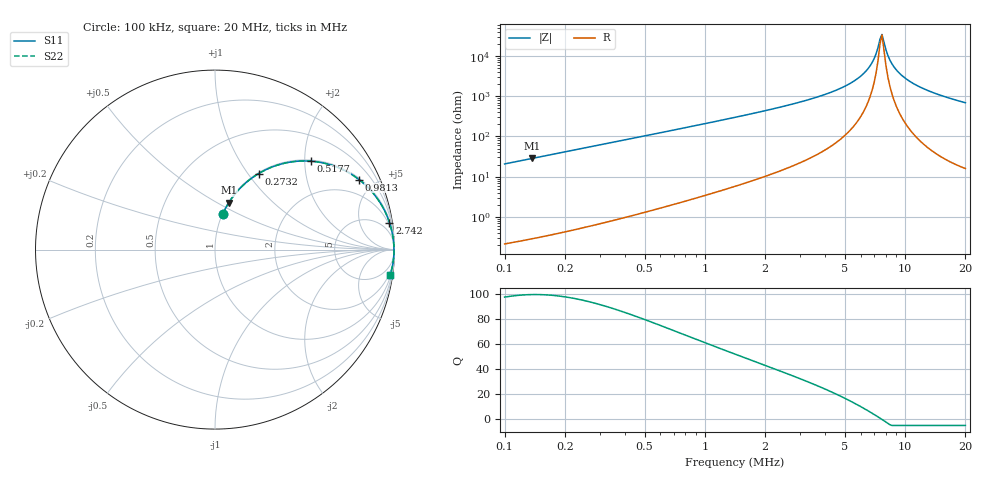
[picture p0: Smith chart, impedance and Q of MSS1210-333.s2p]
# MHz S MA R 50
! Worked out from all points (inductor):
!   233 points, 100 kHz to 20 MHz, reference 50 ohm
!   read as one part in series: L = 33 uH near 102.3 kHz
!   highest Q = 99.7 at 137.7 kHz (marker M1), where L = 32.9 uH
!   self-resonance near 7.491 MHz
!   S11 on the Smith chart (normalised r, x): 100 kHz: 1.00, +0.41; 273.2 kHz: 1.01, +1.13; 517.7 kHz: 1.03, +2.14; 981.3 kHz: 1.07, +4.08; 2.742 MHz: 1, +13; 20 MHz: 1, -14
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0.1  0.2027 77.7  0.9772 -11.7  0.9772 -11.7  0.2027 77.7
0.1376751  0.2734 73.6  0.9592 -15.9  0.9592 -15.9  0.2734 73.6
0.2436751  0.4476 62.8  0.8895 -26.6  0.8895 -26.6  0.4476 62.8
0.2731507  0.4889 60.1  0.8671 -29.3  0.8671 -29.3  0.4889 60.1
0.5177412  0.7255 42.8  0.6791 -46.5  0.6791 -46.5  0.7255 42.8
0.5937753  0.7699 38.9  0.628 -50.3  0.628 -50.3  0.7699 38.9
0.9813485  0.8924 25.9  0.437 -63.2  0.437 -63.2  0.8924 25.9
1.446882  0.9453 18.0  0.3084 -70.9  0.3084 -70.9  0.9453 18.0
2.742482  0.9837 8.8  0.1535 -79.5  0.1535 -79.5  0.9837 8.8
3.446086  0.9897 6.5  0.1125 -81.5  0.1125 -81.5  0.9897 6.5
4.853998  0.9948 3.4  0.06023 -83.3  0.06023 -83.3  0.9948 3.4
6.099327  0.9965 1.7  0.02931 -82.3  0.02931 -82.3  0.9965 1.7
6.531856  0.9968 1.2  0.02041 -80.4  0.02041 -80.4  0.9968 1.2
6.995058  0.997 0.6  0.01168 -74.8  0.01168 -74.8  0.997 0.6
7.491107  0.9971 0.1  0.00379 -40.5  0.00379 -40.5  0.9971 0.1
7.664154  0.9971 -0.0  0.002894 9.3  0.002894 9.3  0.9971 -0.0
8.022333  0.9972 -0.4  0.006954 65.7  0.006954 65.7  0.9972 -0.4
8.397251  0.9971 -0.7  0.01257 76.5  0.01257 76.5  0.9971 -0.7
9.413006  0.9969 -1.6  0.02728 82.7  0.02728 82.7  0.9969 -1.6
11.04475  0.9961 -2.8  0.04869 84.1  0.04869 84.1  0.9961 -2.8
14.19896  0.9936 -4.9  0.08497 83.3  0.08497 83.3  0.9936 -4.9
20  0.9865 -8.2  0.1428 80.5  0.1428 80.5  0.9865 -8.2
